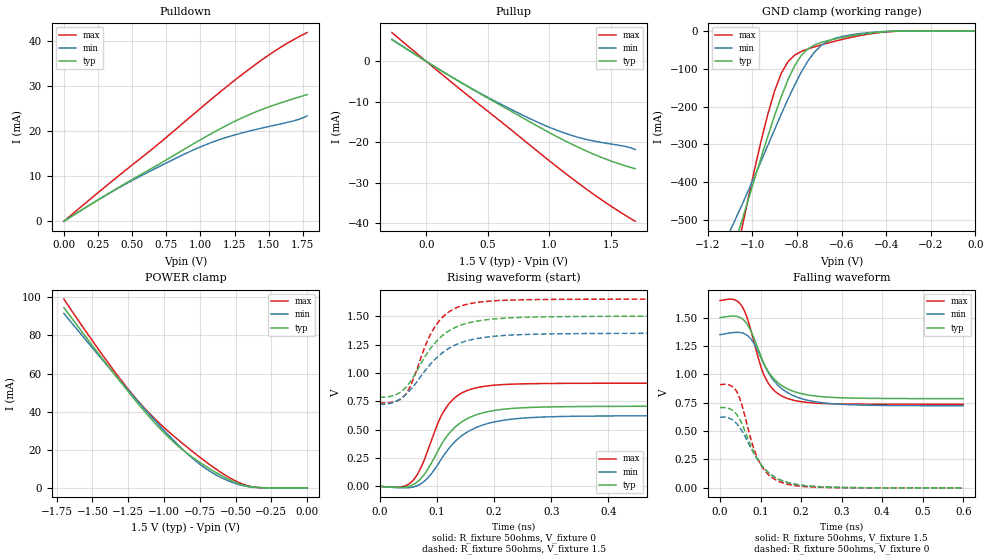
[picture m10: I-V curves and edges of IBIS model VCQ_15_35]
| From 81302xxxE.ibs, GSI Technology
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[Model]   VCQ_15_35
Model_type   Output
Polarity   Non-Inverting
Vmeas =   0.75v
Rref  =   50
|  variable   typ   min   max
C_comp   3.0pF   2.5pF   3.5pF
|  variable   typ   min   max
[Temperature Range]   50   100   0
|  variable   typ   min   max
[Voltage Range]   1.5   1.35   1.65
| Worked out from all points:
|   slope of the pulldown table from 0 to 0.225 V, typ, clamps not added: 52.5 ohm
|   slope of the pullup table from 0 to 0.225 V, typ, clamps not added: 53.7 ohm
|   GND clamp passes 1 mA (typ) near -0.36 V on its own axis
|   POWER clamp passes 1 mA (typ) near -0.42 V on its own axis
|   rising waveform, R_fixture 50ohms, V_fixture 0: 20-80 % time 59.8ps typ, 67.7ps min, 47.5ps max; typ from 0 V to 0.706 V
|   rising waveform, R_fixture 50ohms, V_fixture 1.5: 20-80 % time 62.6ps typ, 70.5ps min, 48.9ps max; typ from 0.786 V to 1.5 V
|   falling waveform, R_fixture 50ohms, V_fixture 1.5: 20-80 % time 62.8ps typ, 71.4ps min, 49.9ps max; typ from 1.5 V to 0.786 V
|   falling waveform, R_fixture 50ohms, V_fixture 0: 20-80 % time 62.8ps typ, 68.3ps min, 50.3ps max; typ from 0.706 V to 0 V
[Pullup]
| V(VDDQ-Vout)   typ   min   max
-280mV    5.393mA    5.499mA    7.154mA
40mV      -756.8uA   -760.1uA   -1.014mA
340mV     -6.266mA   -6.207mA   -8.469mA
620mV     -11.13mA   -10.8mA    -15.22mA
900mV     -15.95mA   -14.97mA   -22.14mA
1.06V     -18.59mA   -17.01mA   -26.03mA
1.22V     -21.03mA   -18.66mA   -29.77mA
1.48V     -24.41mA   -20.34mA   -35.39mA
1.62V     -25.86mA   -21.07mA   -38.13mA
1.7V      -26.56mA   -21.82mA   -39.6mA
[PullDown]
| voltage   typ   min   max
0V        -5.746nA   -11.99nA   -2.475nA
252mV     4.789mA    4.764mA    6.393mA
468mV     8.7mA      8.52mA     11.71mA
684mV     12.45mA    11.93mA    16.95mA
972mV     17.59mA    16.13mA    24.32mA
1.188V    21.2mA     18.59mA    29.75mA
1.314V    23.06mA    19.67mA    32.75mA
1.44V     24.67mA    20.6mA     35.59mA
1.62V     26.59mA    21.82mA    39.19mA
1.71V     27.44mA    22.51mA    40.74mA
1.782V    28.11mA    23.38mA    41.86mA
[POWER Clamp]
|V(VDDQ-Vout)   typ   min   max
-1.7V     94.64mA    91.58mA    99.09mA
-1.428V   67.54mA    66.99mA    69.55mA
-1.224V   48.12mA    49.01mA    49.38mA
-1.122V   38.97mA    40.27mA    40.69mA
-986mV    27.88mA    29.06mA    30.72mA
-816mV    16.83mA    16.48mA    19.99mA
-714mV    11.58mA    10.4mA     14.03mA
-646mV    8.438mA    7.201mA    10.33mA
-544mV    4.31mA     3.482mA    5.399mA
-442mV    1.34mA     1.042mA    1.733mA
-340mV    155.8uA    132.4uA    187.3uA
0V        29.97nA    53.04nA    12.57nA
[GND Clamp]
|(Vout)   typ   min   max
-1.5V     -1.259A    -998.1mA   -1.702A
-1.11V    -621.1mA   -540.5mA   -701.3mA
-1.08V    -564.5mA   -502.7mA   -615.1mA
-1.05V    -506.9mA   -463.9mA   -529.8mA
-930mV    -276.8mA   -301.4mA   -218mA
-900mV    -223mA     -260.1mA   -157.9mA
-870mV    -172.8mA   -219.3mA   -111.5mA
-810mV    -91.52mA   -142.2mA   -63.98mA
-720mV    -36.91mA   -55.08mA   -42.14mA
-630mV    -21.51mA   -20.02mA   -27.42mA
-390mV    -1.861mA   -1.298mA   -2.48mA
0V        -7.463nA   -15.47nA   -3.343nA
[Ramp]
| voltage   typ   min   max
dV/dt_r   0.54/186p   0.48/213p   0.60/209p
dV/dt_f   0.86/129p   0.66/166p   1.07/101p
R_load  =   50ohms
[Rising Waveform]
R_fixture =   50ohms
V_fixture =   0
| Time   V(typ)   V(min)   V(max)
0s        145.8nV    302.9nV    54.13nV
36ps      -8.8mV     -12.42mV   -6.019mV
60ps      19.12mV    -4.075mV   63mV
84ps      151.2mV    74.4mV     316.8mV
102ps     315.4mV    194.9mV    561.2mV
114ps     418.1mV    288.1mV    677.9mV
132ps     524.1mV    397.1mV    784.7mV
162ps     617.5mV    503.3mV    859.9mV
264ps     695.6mV    605.8mV    904.7mV
600ps     706.2mV    622.4mV    909.4mV
[Rising Waveform]
R_fixture =   50ohms
V_fixture =   1.5
V_fixture_min =  1.35
V_fixture_max =  1.65
| Time   V(typ)   V(min)   V(max)
0s        786.4mV    723.5mV    736.6mV
24ps      800.2mV    740.2mV    742.9mV
42ps      853.6mV    793.7mV    790.9mV
54ps      925.8mV    852.8mV    886.8mV
78ps      1.135V     1.011V     1.217V
96ps      1.26V      1.115V     1.401V
120ps     1.368V     1.214V     1.535V
144ps     1.424V     1.27V      1.593V
252ps     1.49V      1.338V     1.644V
600ps     1.5V       1.349V     1.65V
[Falling Waveform]
R_fixture =   50ohms
V_fixture =   1.5
V_fixture_min = 1.35
V_fixture_max = 1.65
| Time   V(typ)   V(min)   V(max)
0s        1.5V       1.35V      1.65V
36ps      1.513V     1.37V      1.657V
54ps      1.492V     1.366V     1.601V
78ps      1.369V     1.304V     1.366V
108ps     1.098V     1.09V      997.7mV
132ps     964.2mV    947.9mV    862.7mV
156ps     892.7mV    864.3mV    802.8mV
204ps     827.6mV    783.1mV    757.5mV
270ps     798.8mV    743.4mV    741.5mV
600ps     786.5mV    723.7mV    736.6mV
[Falling Waveform]
R_fixture =   50ohms
V_fixture =   0
| Time   V(typ)   V(min)   V(max)
0s        706.4mV    622.7mV    909.5mV
24ps      697mV      612.4mV    905.1mV
42ps      643mV      562.9mV    843.6mV
54ps      566.9mV    503.1mV    732.2mV
78ps      355.2mV    339.4mV    406.6mV
90ps      268.5mV    263.7mV    283mV
114ps     151.7mV    153.1mV    137.8mV
144ps     75.73mV    77.58mV    58.34mV
252ps     8.293mV    9.236mV    4.113mV
600ps     23.78uV    56.63uV    4.292uV
